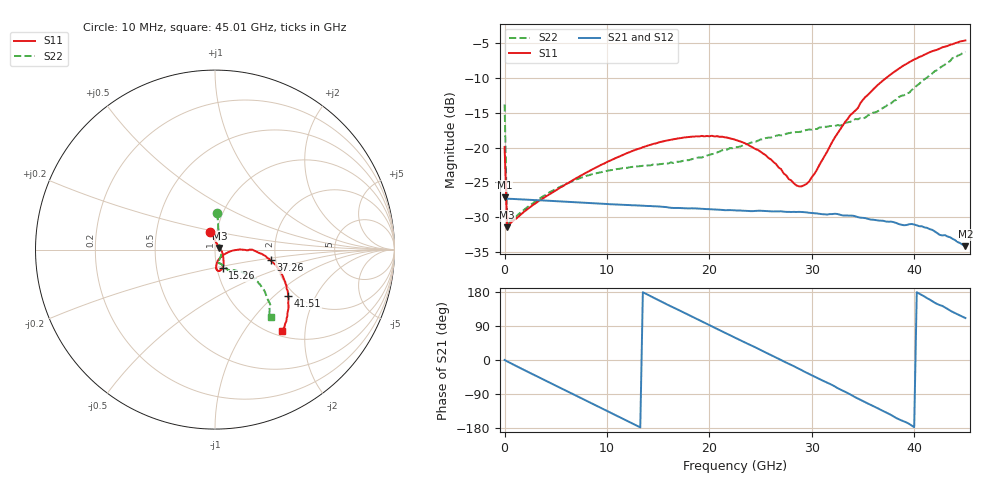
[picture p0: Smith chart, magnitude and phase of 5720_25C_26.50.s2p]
! Device:  ADRF5720
! Description: 0.5dB LSB GaAs MMIC 6-bit Digital Attenuator
! Frequency:  0.000009 -  40 GHz
! Ports:
!	RF1	= Port 1
!	RF2	= Port 2
! Vdd:  3.3 Volt
! Vss:  -3.3 Volt
! Control:  0/3.3 Volt
! State:  26.50 dB attenuation
! Data:  The device was measured using G-S-G Probes on a matrix board.
!  Data was collected using an calibrated 4 port network analyzer.
!  The reference plane for this measurement is at the launchers.
! Note:  Analog Devices supplies this data as a sample of measured data
!  for this product.  Your particular data for this product may vary.
!  Data was taken at 25 degrees C.
!  Analog Devices reserves the right to change this data at anytime.
# GHZ S DB R 45.0
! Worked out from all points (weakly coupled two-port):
!   181 points, 10 MHz to 45.01 GHz, reference 45 ohm
!   highest |S21| = -27.15 dB at 10 MHz (marker M1); lowest = -34.2 dB at 45.01 GHz (marker M2)
!   lowest |S11| = -31.5 dB at 260 MHz (marker M3), VSWR 1.05, Z = 47.3 + j0.872 ohm
!   |S11| at or under -10 dB: start of sweep to 37.28 GHz
!   |S22| runs from -31.3 to -6.2 dB; largest |S21 - S12| = 0.00014
!   S11 on the Smith chart (normalised r, x): 10 MHz: 0.93, +0.18; 15.26 GHz: 1.07, -0.22; 37.26 GHz: 1.88, -0.25; 41.51 GHz: 1.84, -1.24; 45.01 GHz: 1.09, -1.51
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0.01  -19.92 106.4  -27.15 0.1  -27.16 0.1  -13.81 86.3
0.26  -31.47 20.2  -27.35 -3.7  -27.35 -3.8  -31.31 17.3
0.51  -30.97 11.1  -27.36 -7.2  -27.37 -7.2  -30.64 7.1
3.26  -27.77 -17.3  -27.57 -44.4  -27.57 -44.4  -27.48 -34.1
7.76  -23.78 -44.1  -27.92 -104.3  -27.92 -104.3  -24.19 -67.0
12.01  -20.77 -58.5  -28.25 -161.0  -28.25 -161.0  -22.90 -77.1
15.26  -19.18 -67.2  -28.49 154.9  -28.49 155.0  -22.37 -76.2
19.26  -18.33 -77.3  -28.80 101.8  -28.80 101.8  -21.44 -68.6
21.26  -18.44 -82.1  -28.96 75.2  -28.96 75.2  -20.39 -64.7
22.76  -19.00 -85.3  -29.05 55.7  -29.05 55.7  -19.94 -62.2
25.51  -21.10 -85.0  -29.12 19.7  -29.12 19.7  -18.64 -60.4
28.51  -25.45 -58.1  -29.26 -20.0  -29.26 -20.0  -17.77 -58.9
29.51  -25.21 -34.9  -29.33 -33.7  -29.32 -33.7  -17.47 -56.9
30.26  -23.79 -18.5  -29.43 -43.5  -29.43 -43.5  -17.32 -56.6
33.26  -16.32 -0.0  -29.76 -83.8  -29.76 -83.8  -16.45 -50.1
35.26  -12.71 -2.7  -30.15 -111.8  -30.14 -111.7  -15.66 -45.1
37.26  -10.02 -11.0  -30.63 -138.6  -30.64 -138.6  -14.05 -39.5
37.76  -9.44 -13.3  -30.64 -145.2  -30.64 -145.2  -13.64 -38.5
39.51  -7.75 -21.9  -31.02 -168.5  -31.02 -168.4  -12.14 -37.9
41.51  -6.31 -32.3  -31.71 159.8  -31.73 159.8  -9.62 -38.5
43.76  -5.15 -43.8  -33.11 126.9  -33.11 126.9  -7.12 -45.2
45.01  -4.61 -50.7  -34.17 110.8  -34.14 110.8  -6.23 -50.6
